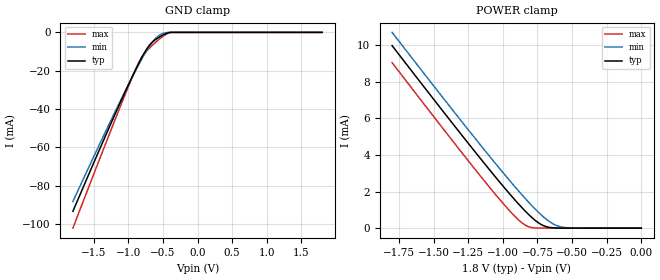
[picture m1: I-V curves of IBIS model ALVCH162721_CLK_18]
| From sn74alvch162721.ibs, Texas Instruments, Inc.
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[Model]   ALVCH162721_CLK_18
Model_type  Input
Vinl = 0.5775
Vinh = 1.2675
| variable   typ   min   max
C_comp   1.90pF   1.76pF   2.20pF
[Temperature Range]   40   100   -40
| Ambient temperature   25   85   -40
[Voltage range]   1.8   1.65   1.95
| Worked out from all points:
|   GND clamp passes 1 mA (typ) near -0.48 V on its own axis
|   POWER clamp passes 1 mA (typ) near -0.85 V on its own axis
[GND Clamp]
| ALVCH162721_CLK_18
|   Voltage   I(typ)   I(min)   I(max)
-1.8V     -93.3mA    -88.19mA   -102.1mA
-1.235V   -46.25mA   -44.72mA   -49.56mA
-1V       -27.5mA    -27.4mA    -28.37mA
-875mV    -18.04mA   -18.61mA   -17.75mA
-795mV    -12.45mA   -13.28mA   -12.37mA
-700mV    -6.981mA   -7.539mA   -8.412mA
-615mV    -3.968mA   -3.483mA   -5.497mA
-535mV    -2.13mA    -1.195mA   -3.054mA
-445mV    -515.8uA   -125.4uA   -861.2uA
-375mV    -85.17nA   -8.524uA   -4.38uA
1.8V      24.55pA    142.2pA    23.4pA
[POWER Clamp]
| ALVCH162721_CLK_18
|   Voltage   I(typ)   I(min)   I(max)
-1.8V     9.965mA    10.69mA    9.037mA
-1.38V    5.878mA    6.614mA    4.929mA
-1.105V   3.269mA    4.008mA    2.314mA
-940mV    1.776mA    2.501mA    856.4uA
-885mV    1.307mA    2.018mA    440uA
-845mV    982.9uA    1.676mA    200.1uA
-795mV    611.2uA    1.266mA    38.41uA
-715mV    166.7uA    670.1uA    941.7nA
-645mV    22.22uA    268.3uA    31.48nA
-585mV    2.717uA    77.14uA    1.709nA
-485mV    73.51nA    4.604uA    18.27pA
-16.28fV  3.325pA    5.122pA    3.398pA
